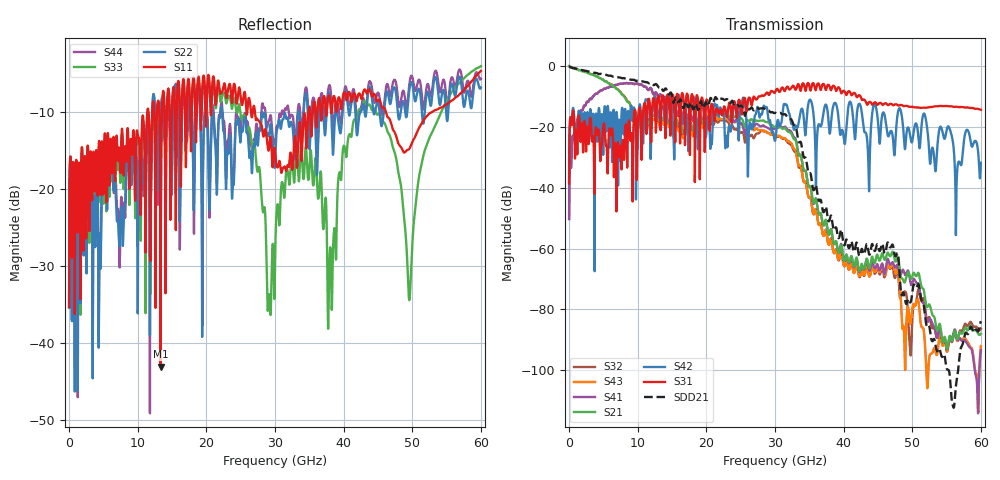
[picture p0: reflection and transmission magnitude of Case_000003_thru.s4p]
! Info: Touchstone file created by circ.  Input file=CasetestDOE_NRZ_template_000003.circ
# Hz S RI R 50
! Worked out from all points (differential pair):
!   6000 points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, 10 MHz to 60 GHz, reference 50 ohm
!   strongest paths, dB at 10 MHz, 15.01 GHz, 30.01 GHz, 45.01 GHz, 60 GHz:
!     S31: -38.6, -9.5, -8.7, -12.7, -14.4
!     S42: -38.6, -14.8, -24.6, -18.3, -31.8
!     S21: -0.1, -20.7, -20.0, -62.6, -88.0
!     S41: -50.3, -12.2, -20.4, -65.8, -93.3
!     S43: -0.1, -20.6, -22.8, -66.2, -92.0
!     S32: -50.3, -13.2, -22.8, -66.6, -86.3
!   taken as a pair (ports 1,3 in; 2,4 out), SDD21 dB: -0.1, -9.9, -15.4, -59.3, -83.8
!   lowest |S11| = -43.1 dB at 13.34 GHz (marker M1), VSWR 1.01, Z = 50.5 + j0.49 ohm
!   |S11| at or under -10 dB: start of sweep to 11.4 GHz; 27.08 GHz to 34.86 GHz (7.783 GHz wide, 25.1 % of centre); 46.18 GHz to 52.83 GHz (6.656 GHz wide, 13.4 % of centre)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
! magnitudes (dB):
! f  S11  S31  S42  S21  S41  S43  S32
! 10 MHz  -35.3  -38.6  -38.6  -0.1  -50.3  -0.1  -50.3
! 2.81 GHz  -15.8  -24.3  -19.8  -2.4  -11.8  -2.3  -11.8
! 13.34 GHz  -43.1  -21.1  -14.1  -17.8  -9.4  -18.9  -9.5
! 31.59 GHz  -17.6  -7.5  -12.7  -20.8  -20.2  -24.0  -24.3
! 40.09 GHz  -7.4  -8.3  -25.0  -64.1  -63.9  -65.6  -65.8
! 49.59 GHz  -14.7  -13.4  -21.6  -68.6  -69.4  -83.8  -89.9
! 60 GHz  -4.6  -14.4  -31.8  -88.0  -93.3  -92.0  -86.3
